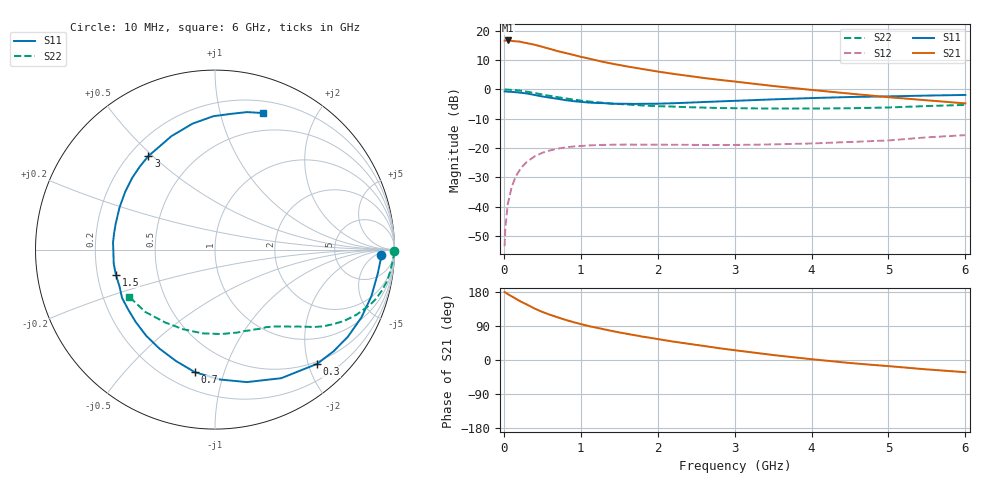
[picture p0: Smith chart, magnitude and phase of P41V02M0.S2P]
! SIEMENS Small Signal Semiconductors
! BFP182
! Si NPN RF Bipolar Junction Transistor in SOT143
! VCE = 1 V  IC = 2 mA
! Common Emitter S-Parameters:  March  1996
# GHz  S  MA  R  50
!  f  S11  S21  S12  S22
! GHz  MAG  ANG  MAG  ANG  MAG  ANG  MAG  ANG
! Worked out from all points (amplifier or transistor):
!   36 points, 10 MHz to 6 GHz, reference 50 ohm
!   highest |S21| = 16.8 dB at 50 MHz (marker M1)
!   |S21| within 3 dB of that: start of sweep to 615.2 MHz
!   unconditionally stable (mu >= 1): 2.104 GHz to end of sweep
!   at 250 MHz: K = 0.13, MSG = 21.1 dB, |S12| = -26.1 dB
!   at 1.4 GHz: K = 0.70, MSG = 13.9 dB, |S12| = -18.9 dB
!   at 6 GHz: K = 1.09, MAG = 3.6 dB, |S12| = -15.6 dB
!   S11 on the Smith chart (normalised r, x): 10 MHz: 23, -9; 300 MHz: 0.46, -2.15; 700 MHz: 0.31, -0.80; 1.5 GHz: 0.28, -0.11; 3 GHz: 0.27, +0.48; 6 GHz: 0.31, +1.36
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0.01  0.9272 -1.7  6.83 179.2  0.0021 87.2  0.9959 -0.6
0.02  0.925 -3.3  6.83 178.3  0.0043 87.3  0.9982 -1.4
0.05  0.9166 -8.4  6.88 174.1  0.0108 87.7  0.9925 -3.5
0.1  0.9092 -16.6  6.76 168.2  0.021 80.3  0.9842 -7.0
0.2  0.8853 -33.3  6.599 156.5  0.041 70.8  0.958 -13.7
0.3  0.8536 -48.3  6.192 146.3  0.0581 62.1  0.9167 -19.6
0.4  0.8057 -62.8  5.818 135.7  0.0717 54.8  0.8692 -24.6
0.5  0.7592 -76.5  5.361 126.9  0.0827 47.6  0.8209 -29.0
0.6  0.724 -88.0  4.937 119.4  0.0909 42.2  0.7767 -32.4
0.7  0.6919 -99.4  4.516 112.5  0.0975 37.6  0.7395 -35.3
0.8  0.6575 -109.4  4.209 106.0  0.1021 33.3  0.7045 -37.7
0.9  0.6323 -119.4  3.912 100.2  0.106 29.9  0.6734 -39.7
1.1  0.5981 -137.5  3.388 89.7  0.1104 24.2  0.6248 -43.3
1.3  0.5839 -152.4  2.945 81.1  0.1129 19.5  0.5902 -46.5
1.5  0.5698 -165.9  2.622 72.8  0.1141 16.2  0.5643 -49.3
1.8  0.5695 176.1  2.237 61.8  0.114 13.2  0.5337 -53.4
2.2  0.5815 156.1  1.851 48.7  0.1136 10.1  0.5098 -59.7
3  0.6395 125.5  1.367 25.8  0.1127 8.6  0.4787 -74.9
3.5  0.6772 111.0  1.147 13.1  0.1152 9.3  0.4716 -86.0
4.5  0.7433 90.7  0.849 -8.0  0.1267 11.3  0.4778 -111.7
5.5  0.7865 76.9  0.653 -24.8  0.1521 11.7  0.5209 -138.2
6  0.8062 70.7  0.578 -32.2  0.1657 9.0  0.5449 -151.0
